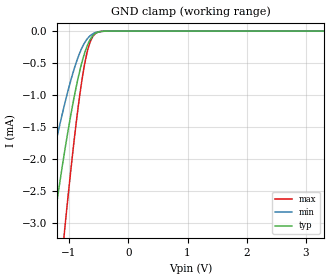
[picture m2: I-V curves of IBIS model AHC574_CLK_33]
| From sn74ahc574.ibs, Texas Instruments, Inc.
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[Model]   AHC574_CLK_33
Model_type  Input
Vinl = 0.9
Vinh = 2.1
| variable   typ   min   max
C_comp   0.90pF   0.77pF   1.02pF
[Temperature Range]   40   100   -40
| Ambient temperature   25   85   -40
[Voltage range]   3.3   3   3.6
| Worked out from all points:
|   GND clamp passes 1 mA (typ) near -0.91 V on its own axis
[GND Clamp]
| AHC574_CLK_33
|   Voltage   I(typ)   I(min)   I(max)
-3.3V     -21.16mA   -13.85mA   -28.81mA
-1.52V    -4.862mA   -3.106mA   -7.679mA
-1.28V    -3.16mA    -1.987mA   -5.134mA
-1.1V     -2.029mA   -1.24mA    -3.353mA
-1.07V    -1.855mA   -1.126mA   -3.072mA
-905mV    -991.3uA   -566.5uA   -1.636mA
-835mV    -686uA     -378.6uA   -1.111mA
-780mV    -480.2uA   -258.4uA   -753.3uA
-690mV    -222.9uA   -118.8uA   -314.3uA
-590mV    -64.59uA   -38.14uA   -73.95uA
-375mV    -1.358uA   -994.5nA   -683.1nA
3.3V      3.761nA    612.9pA    18.13nA
